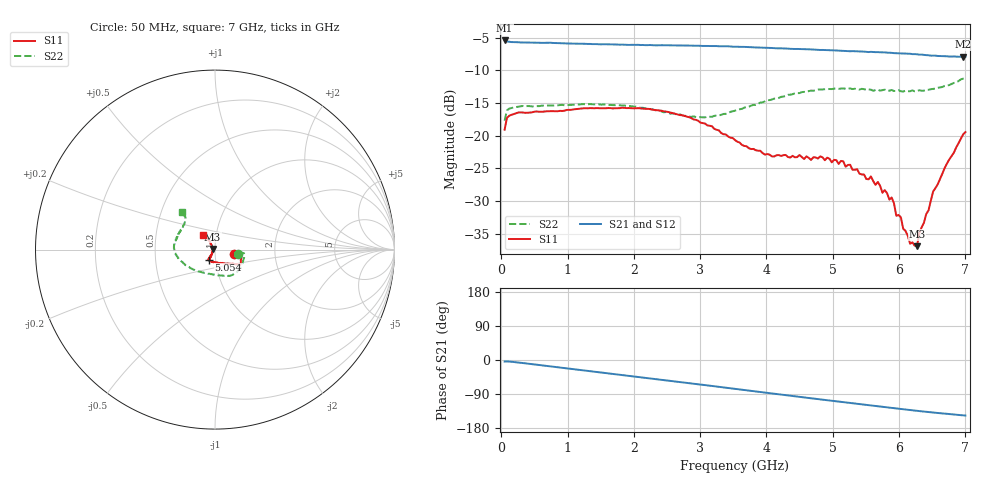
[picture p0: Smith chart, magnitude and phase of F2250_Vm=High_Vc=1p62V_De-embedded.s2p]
! Integrated Device Technology
! Corporate Headquarters
! 6024 Silver Creek Valley Road
! San Jose, CA 95138  USA
! Phone:  1-408-284-8200
! Toll Free:  1-800-223-1366
! Webpage:  http://www.idt.com/
! Timing and RF Division
! 515 Groton Road, Suite 102
! Westford, MA 01886-6024
! Device:  F2250
! Description: Voltage Variable RF Attenuator
! Frequency:  50.0 -  6000.00 MHz
! Package:  3x3 mm Thin QFN Plastic Package: 16 pin
! Ports:  2 RF, 3 DC
!  Pin  1  = GND
!  Pin  2  = NC
!  Pin  3  = RF1  = Port 1
!  Pin  4  = NC
!  Pin  5  = GND
!  Pin  6  = GND
!  Pin  7  = GND
!  Pin  8  = GND
!  Pin  9  = NC
!  Pin 10  = RF2  = Port 2
!  Pin 11  = NC
!  Pin 12  = GND
!  Pin 13  = GND
!  Pin 14  = VCNTRL
!  Pin 15  = VDD
!  Pin 16  = VMODE
! Vcntrl:  1.620 Volts
! Vmode:  +3.300 Volts
! Vdd:  +3.30  Volts
! Current:  1.326 mA
! Data:  The device was measured on a the F2250 evaluation board which has
!  individual transmission lines to the RF pins.  Data was collected
!  using a calibrated network analyzer.  The evaluation board was
!  de-embedded using a TRL calibration technique.
!  The reference plane is the edge of the package pin.
! Misc:  SN 10
!  Action Tracker AT0258
! Date Measured:  2014-11-26
! Date:  2015-10-15  MJV
! Note:
!  Integrated Device Technology supplies this data as a sample of measured
!  data at the package pin for this product.  Your particular data for this
!  product may vary.
!  Data was taken at 25 degrees C.
!  Integrated Device Technology reserves the right to change this data at anytime.
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# GHz S dB R 50
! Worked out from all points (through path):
!   201 points, 50 MHz to 7 GHz, reference 50 ohm
!   highest |S21| = -5.43 dB at 50 MHz (marker M1); lowest = -7.9 dB at 6.965 GHz (marker M2)
!   group delay of S21, straight-line fit = 58.8 ps
!   lowest |S11| = -36.9 dB at 6.27 GHz (marker M3), VSWR 1.03, Z = 48.6 + j0.348 ohm
!   |S11| at or under -10 dB: start of sweep to end of sweep
!   |S22| runs from -17.7 to -11.1 dB; largest |S21 - S12| = 0.003
!   S11 on the Smith chart (normalised r, x): 50 MHz: 1.24, -0.07; 5.054 GHz: 0.93, -0.10; 7 GHz: 0.86, +0.14
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0.05  -19.08 -13.6  -5.43 -4.1  -5.42 -4.0  -17.70 -11.9
0.08475  -17.29 -7.4  -5.58 -3.8  -5.57 -3.8  -16.13 -7.5
0.2585  -16.44 -8.0  -5.70 -6.7  -5.73 -6.7  -15.57 -11.5
1.2315  -15.82 -26.2  -5.94 -27.4  -5.95 -27.4  -15.17 -42.9
2.37825  -16.12 -32.3  -6.16 -51.2  -6.16 -51.2  -16.14 -70.7
2.969  -17.71 -37.5  -6.24 -63.9  -6.24 -64.0  -17.22 -96.9
3.525  -20.67 -55.6  -6.38 -76.1  -6.38 -76.2  -16.18 -129.7
4.081  -23.16 -88.7  -6.58 -88.3  -6.57 -88.3  -14.47 -155.3
4.7065  -23.31 -117.7  -6.82 -101.7  -6.82 -101.7  -13.12 -173.9
5.054  -23.75 -120.9  -6.96 -109.1  -6.95 -109.1  -12.77 177.7
5.57525  -26.24 -123.3  -7.17 -119.8  -7.16 -119.9  -12.97 165.5
5.85325  -29.78 -125.2  -7.31 -125.6  -7.31 -125.7  -13.12 156.9
5.888  -29.46 -127.9  -7.32 -126.4  -7.30 -126.5  -13.00 157.0
5.9575  -32.25 -125.2  -7.38 -127.7  -7.35 -127.9  -13.17 154.1
6.027  -32.50 -135.0  -7.41 -129.2  -7.40 -129.3  -13.20 152.8
6.166  -36.55 -157.3  -7.46 -132.0  -7.48 -132.1  -13.20 147.6
6.27025  -36.91 165.5  -7.55 -134.1  -7.55 -134.2  -13.19 144.2
6.305  -34.87 149.2  -7.60 -134.8  -7.59 -134.9  -13.04 143.2
6.444  -31.43 131.0  -7.69 -137.4  -7.69 -137.5  -12.97 139.1
6.5135  -28.55 126.2  -7.76 -138.6  -7.74 -138.8  -12.84 136.9
6.96525  -19.81 128.7  -7.93 -146.1  -7.97 -146.1  -11.28 131.8
7  -19.45 128.9  -7.93 -146.6  -7.97 -146.7  -11.12 131.0
